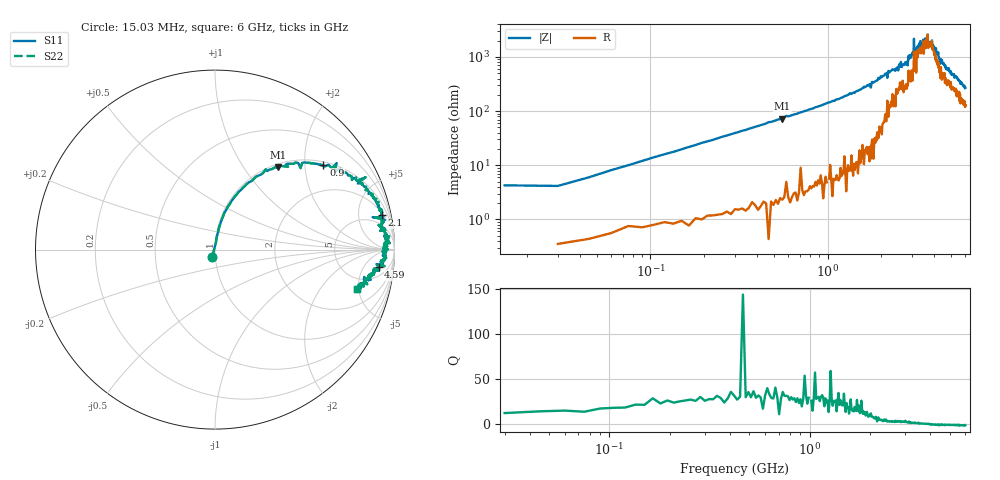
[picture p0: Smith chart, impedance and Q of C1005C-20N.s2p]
!	Network	Analyzer	HP8753E.07.74:	Oct	30	2002	Serial	No.	JP38451487
!	Hewlett-Packard
!	7	Sep	2009	8:52:36
!	Frequency	S11	S21	S12	S22
#	HZ	S	RI	R	50
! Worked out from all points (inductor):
!   400 points, 15.03 MHz to 6 GHz, reference 50 ohm
!   read as one part in series: L = 21.2 nH near 45.03 MHz
!   highest Q = 31.4 at 555 MHz (marker M1), where L = 20.8 nH
!   self-resonance near 3.524 GHz
!   S11 on the Smith chart (normalised r, x): 15.03 MHz: 0.97, -0.08; 900 MHz: 1.09, +2.49; 2.1 GHz: 2.42, +9.20; 4.59 GHz: 9, -11; 6 GHz: 3.56, -4.74
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1.502992e7  -0.0154 -0.0397  1.02 0.0397  1.02 0.0397  -0.0154 -0.0397
1.95029e8  0.0708 0.238  0.929 -0.238  0.929 -0.238  0.0708 0.238
5.550272e8  0.349 0.461  0.651 -0.461  0.651 -0.461  0.349 0.461
9.000255e8  0.604 0.471  0.396 -0.471  0.396 -0.471  0.604 0.471
1.020025e9  0.67 0.451  0.33 -0.451  0.33 -0.451  0.67 0.451
2.01002e9  0.924 0.213  0.0759 -0.213  0.0759 -0.213  0.924 0.213
2.10002e9  0.929 0.191  0.0712 -0.191  0.0712 -0.191  0.929 0.191
2.835016e9  0.928 0.113  0.0717 -0.113  0.0717 -0.113  0.928 0.113
3.015015e9  0.97 0.0746  0.0301 -0.0746  0.0301 -0.0746  0.97 0.0746
3.060015e9  0.956 0.063  0.0441 -0.063  0.0441 -0.063  0.956 0.063
3.075015e9  0.973 0.0355  0.0274 -0.0355  0.0274 -0.0355  0.973 0.0355
3.105014e9  0.953 0.0692  0.0472 -0.0692  0.0472 -0.0692  0.953 0.0692
3.165014e9  0.944 0.0777  0.0565 -0.0777  0.0565 -0.0777  0.944 0.0777
3.345013e9  0.968 0.037  0.0324 -0.037  0.0324 -0.037  0.968 0.037
3.555012e9  0.96 0.0175  0.0399 -0.0175  0.0399 -0.0175  0.96 0.0175
3.585012e9  0.939 0.0146  0.0611 -0.0146  0.0611 -0.0146  0.939 0.0146
3.675012e9  0.963 0.00128  0.037 -0.00128  0.037 -0.00128  0.963 0.00128
3.705011e9  0.937 0.00476  0.0628 -0.00476  0.0628 -0.00476  0.937 0.00476
4.00501e9  0.952 -0.0421  0.0484 0.0421  0.0484 0.0421  0.952 -0.0421
4.590007e9  0.912 -0.0969  0.0876 0.0969  0.0876 0.0969  0.912 -0.0969
5.010005e9  0.879 -0.13  0.121 0.13  0.121 0.13  0.879 -0.13
6e9  0.789 -0.219  0.211 0.219  0.211 0.219  0.789 -0.219
